FUNCTION_BLOCK "Stato Celle"
TITLE =
VERSION : 0.1


VAR_INPUT
  Start : BOOL ;
  TestingCell1 : BOOL ;
  TestingCell2 : BOOL ;
  TestingCell3 : BOOL ;
  TestingCell4 : BOOL ;
  TestingCell5 : BOOL ;
  TestingCell6 : BOOL ;
  STS_Bell : BOOL ;
END_VAR
VAR_OUTPUT
  CellStatus : ARRAY  [0 .. 7 ] OF BOOL ;
  Stati : ARRAY  [0 .. 10 ] OF INT ;
END_VAR
VAR
  Cell1_NotOK : BOOL ;
  Cell2_NotOK : BOOL ;
  Cell3_NotOK : BOOL ;
  Cell4_NotOK : BOOL ;
  Cell5_NotOK : BOOL ;
  Cell6_NotOK : BOOL ;
  bell_edge : BOOL ;
  Cell1_Tested : BOOL ;
  Cell2_Tested : BOOL ;
  Cell3_Tested : BOOL ;
  Cell4_Tested : BOOL ;
  Cell5_Tested : BOOL ;
  Cell6_Tested : BOOL ;
END_VAR
BEGIN
NETWORK
TITLE =Reset ad inizio ciclo
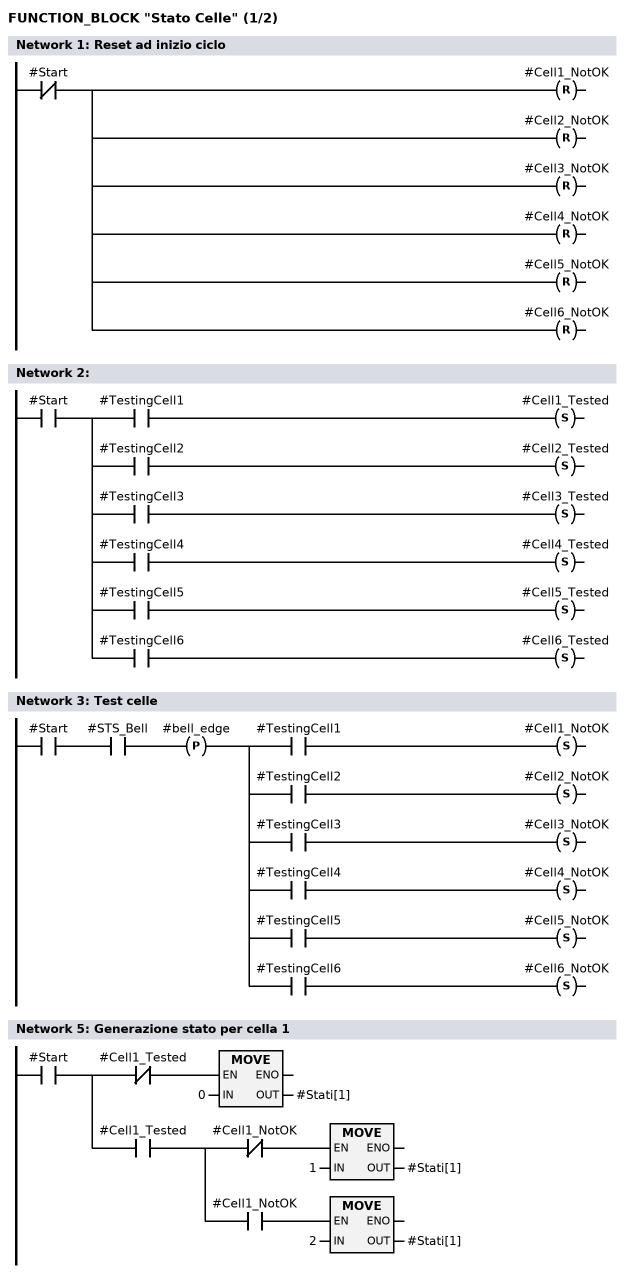
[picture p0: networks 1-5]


      UN    #Start;
      R     #Cell1_NotOK;
      R     #Cell2_NotOK;
      R     #Cell3_NotOK;
      R     #Cell4_NotOK;
      R     #Cell5_NotOK;
      R     #Cell6_NotOK;

NETWORK
TITLE =

      U     #Start;
      =     L      0.0;
      U     L      0.0;
      U     #TestingCell1;
      S     #Cell1_Tested;
      U     L      0.0;
      U     #TestingCell2;
      S     #Cell2_Tested;
      U     L      0.0;
      U     #TestingCell3;
      S     #Cell3_Tested;
      U     L      0.0;
      U     #TestingCell4;
      S     #Cell4_Tested;
      U     L      0.0;
      U     #TestingCell5;
      S     #Cell5_Tested;
      U     L      0.0;
      U     #TestingCell6;
      S     #Cell6_Tested;
NETWORK
TITLE =Test celle

      U     #Start;
      U     #STS_Bell;
      FP    #bell_edge;
      =     L      0.0;
      U     L      0.0;
      U     #TestingCell1;
      S     #Cell1_NotOK;
      U     L      0.0;
      U     #TestingCell2;
      S     #Cell2_NotOK;
      U     L      0.0;
      U     #TestingCell3;
      S     #Cell3_NotOK;
      U     L      0.0;
      U     #TestingCell4;
      S     #Cell4_NotOK;
      U     L      0.0;
      U     #TestingCell5;
      S     #Cell5_NotOK;
      U     L      0.0;
      U     #TestingCell6;
      S     #Cell6_NotOK;
NETWORK
TITLE =
//Stati dipendenti dal tipo di controllo:
//
//0--> cella non ancora controllata
//1--> cella in errore
//3--> cella buona
NETWORK
TITLE =Generazione stato per cella 1

      U     #Start;
      =     L      0.0;
      U     L      0.0;
      UN    #Cell1_Tested;
      SPBNB _001;
      L     0;
      T     #Stati[1];
_001: NOP   0;
      U     L      0.0;
      U     #Cell1_Tested;
      =     L      0.1;
      U     L      0.1;
      UN    #Cell1_NotOK;
      SPBNB _002;
      L     1;
      T     #Stati[1];
_002: NOP   0;
      U     L      0.1;
      U     #Cell1_NotOK;
      SPBNB _003;
      L     2;
      T     #Stati[1];
_003: NOP   0;
NETWORK
TITLE =Generazione stati per cella 2
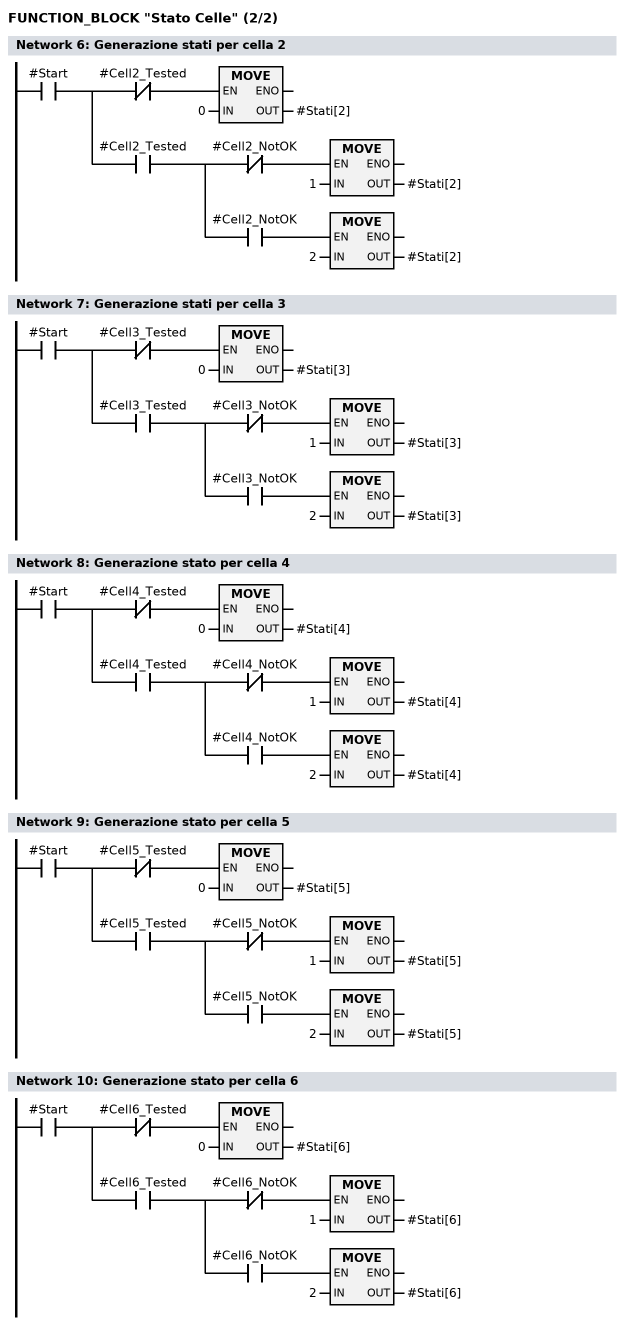
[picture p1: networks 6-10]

      U     #Start;
      =     L      0.0;
      U     L      0.0;
      UN    #Cell2_Tested;
      SPBNB _004;
      L     0;
      T     #Stati[2];
_004: NOP   0;
      U     L      0.0;
      U     #Cell2_Tested;
      =     L      0.1;
      U     L      0.1;
      UN    #Cell2_NotOK;
      SPBNB _005;
      L     1;
      T     #Stati[2];
_005: NOP   0;
      U     L      0.1;
      U     #Cell2_NotOK;
      SPBNB _006;
      L     2;
      T     #Stati[2];
_006: NOP   0;
NETWORK
TITLE =Generazione stati per cella 3

      U     #Start;
      =     L      0.0;
      U     L      0.0;
      UN    #Cell3_Tested;
      SPBNB _007;
      L     0;
      T     #Stati[3];
_007: NOP   0;
      U     L      0.0;
      U     #Cell3_Tested;
      =     L      0.1;
      U     L      0.1;
      UN    #Cell3_NotOK;
      SPBNB _008;
      L     1;
      T     #Stati[3];
_008: NOP   0;
      U     L      0.1;
      U     #Cell3_NotOK;
      SPBNB _009;
      L     2;
      T     #Stati[3];
_009: NOP   0;
NETWORK
TITLE =Generazione stato per cella 4

      U     #Start;
      =     L      0.0;
      U     L      0.0;
      UN    #Cell4_Tested;
      SPBNB _00a;
      L     0;
      T     #Stati[4];
_00a: NOP   0;
      U     L      0.0;
      U     #Cell4_Tested;
      =     L      0.1;
      U     L      0.1;
      UN    #Cell4_NotOK;
      SPBNB _00b;
      L     1;
      T     #Stati[4];
_00b: NOP   0;
      U     L      0.1;
      U     #Cell4_NotOK;
      SPBNB _00c;
      L     2;
      T     #Stati[4];
_00c: NOP   0;
NETWORK
TITLE =Generazione stato per cella 5

      U     #Start;
      =     L      0.0;
      U     L      0.0;
      UN    #Cell5_Tested;
      SPBNB _00d;
      L     0;
      T     #Stati[5];
_00d: NOP   0;
      U     L      0.0;
      U     #Cell5_Tested;
      =     L      0.1;
      U     L      0.1;
      UN    #Cell5_NotOK;
      SPBNB _00e;
      L     1;
      T     #Stati[5];
_00e: NOP   0;
      U     L      0.1;
      U     #Cell5_NotOK;
      SPBNB _00f;
      L     2;
      T     #Stati[5];
_00f: NOP   0;
NETWORK
TITLE =Generazione stato per cella 6

      U     #Start;
      =     L      0.0;
      U     L      0.0;
      UN    #Cell6_Tested;
      SPBNB _010;
      L     0;
      T     #Stati[6];
_010: NOP   0;
      U     L      0.0;
      U     #Cell6_Tested;
      =     L      0.1;
      U     L      0.1;
      UN    #Cell6_NotOK;
      SPBNB _011;
      L     1;
      T     #Stati[6];
_011: NOP   0;
      U     L      0.1;
      U     #Cell6_NotOK;
      SPBNB _012;
      L     2;
      T     #Stati[6];
_012: NOP   0;
END_FUNCTION_BLOCK

